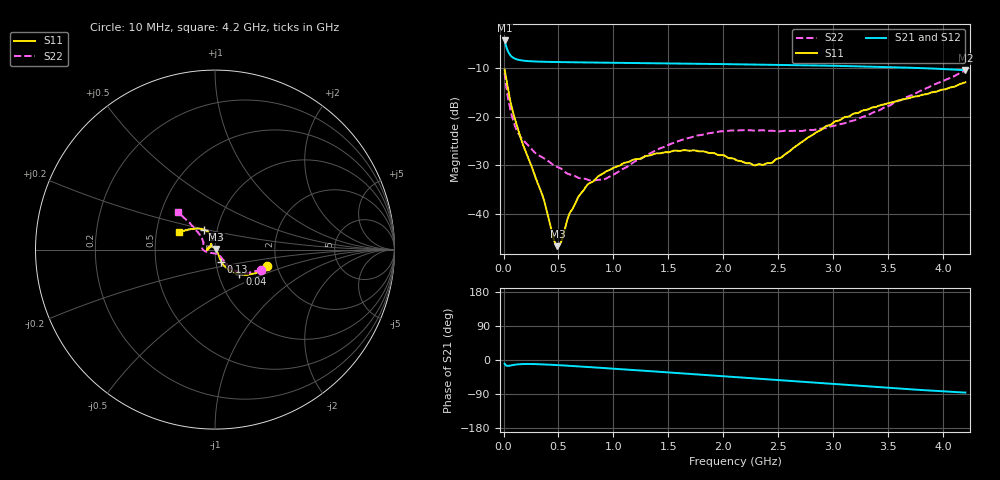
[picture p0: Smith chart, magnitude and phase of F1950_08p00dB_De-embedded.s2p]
! Integrated Device Technology
! Corporate Headquarters
! 6024 Silver Creek Valley Road
! San Jose, CA 95138  USA
! Phone:  1-408-284-8200
! Toll Free:  1-800-223-1366
! Webpage:  http://www.idt.com/
! Timing and RF Division
! 515 Groton Road, Suite 102
! Westford, MA 01886-6024
! Device:  F1950
! Description: 7-bit 0.25 dB Digital Step Attenuator
! Frequency:  150.0 -  4000.00 MHz
! Package:  4x4 mm Thin QFN Plastic Package: 24 pin
! Ports:  2 RF, 12 DC
!  Pin  1  = D0
!  Pin  2  = VDD
!  Pin  3  = Vmode
!  Pin  4  = GND
!  Pin  5  = RF1  =  Port 1
!  Pin  6  = GND
!  Pin  7  = GND
!  Pin  8  = GND
!  Pin  9  = GND
!  Pin 10  = GND
!  Pin 11  = GND
!  Pin 12  = GND
!  Pin 13  = GND
!  Pin 14  = RF2  =  Port 2
!  Pin 15  = GND
!  Pin 16  = LE
!  Pin 17  = CLK
!  Pin 18  = DATE
!  Pin 19  = D6
!  Pin 20  = D5
!  Pin 21  = D4
!  Pin 22  = D3
!  Pin 23  = D2
!  Pin 24  = D1
! State:  32
! Atten State:  8.00 dB
! Voltage:  +5.00 Volts
! Current:  Not Measured mA
! Data:  The device was measured on a the F195X evaluation board which has
!  individual transmission lines to the RF pins.  Data was collected
!  using a calibrated network analyzer.  The evaluation board was
!  de-embedded using a TRL calibration technique.
!  The reference plane is the edge of the package pin.
! Misc:  Board 2019
!  Action Tracker AT0250
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# GHz S dB R 50
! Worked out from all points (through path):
!   420 points, 10 MHz to 4.2 GHz, reference 50 ohm
!   highest |S21| = -4.43 dB at 10 MHz (marker M1); lowest = -10.5 dB at 4.2 GHz (marker M2)
!   group delay of S21, straight-line fit = 53.9 ps
!   lowest |S11| = -46.5 dB at 490 MHz (marker M3), VSWR 1.01, Z = 50.4 + j0.313 ohm
!   |S11| at or under -10 dB: start of sweep to end of sweep
!   |S22| runs from -33.1 to -10.6 dB; largest |S21 - S12| = 0.00046
!   S11 on the Smith chart (normalised r, x): 10 MHz: 1.77, -0.35; 40 MHz: 1.26, -0.36; 130 MHz: 1.06, -0.14; 3.4 GHz: 0.86, +0.20; 4.2 GHz: 0.65, +0.14
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0.01  -10.39 -17.4  -4.43 -9.9  -4.43 -9.9  -11.03 -23.6
0.04  -14.30 -45.3  -6.61 -15.5  -6.61 -15.5  -16.10 -47.2
0.08  -18.57 -58.4  -7.84 -13.6  -7.84 -13.6  -20.20 -51.7
0.13  -22.46 -62.3  -8.36 -11.5  -8.36 -11.5  -23.27 -51.0
0.27  -31.11 -54.3  -8.72 -10.7  -8.72 -10.7  -27.01 -52.2
0.35  -35.85 -43.3  -8.79 -11.5  -8.78 -11.5  -28.28 -54.8
0.45  -44.51 -4.3  -8.84 -12.9  -8.84 -12.8  -29.85 -58.0
0.49  -46.50 41.1  -8.85 -13.5  -8.85 -13.5  -30.31 -61.5
0.53  -45.31 77.7  -8.87 -14.1  -8.87 -14.2  -30.74 -62.7
0.6  -39.84 108.4  -8.89 -15.4  -8.89 -15.4  -31.82 -70.1
0.71  -35.61 124.4  -8.92 -17.4  -8.92 -17.4  -32.66 -83.0
0.93  -31.27 142.5  -8.99 -21.6  -8.98 -21.6  -32.71 -117.8
1.41  -27.53 171.2  -9.11 -31.0  -9.11 -31.0  -26.61 -163.7
1.74  -26.92 -178.5  -9.20 -37.6  -9.20 -37.6  -23.99 -176.1
2.11  -28.80 175.1  -9.31 -45.1  -9.31 -45.1  -22.86 173.7
2.28  -29.97 157.4  -9.36 -48.5  -9.36 -48.6  -22.87 169.3
2.43  -29.52 136.7  -9.41 -51.5  -9.40 -51.5  -22.90 165.1
2.81  -23.76 108.1  -9.53 -59.4  -9.53 -59.4  -22.75 151.2
3.1  -20.13 110.4  -9.65 -65.4  -9.65 -65.4  -21.38 142.7
3.4  -17.91 118.9  -9.81 -71.5  -9.81 -71.5  -18.89 136.4
3.51  -17.19 123.2  -9.88 -73.6  -9.87 -73.7  -17.75 135.0
4.2  -13.00 153.4  -10.54 -85.9  -10.53 -86.0  -10.58 134.7
